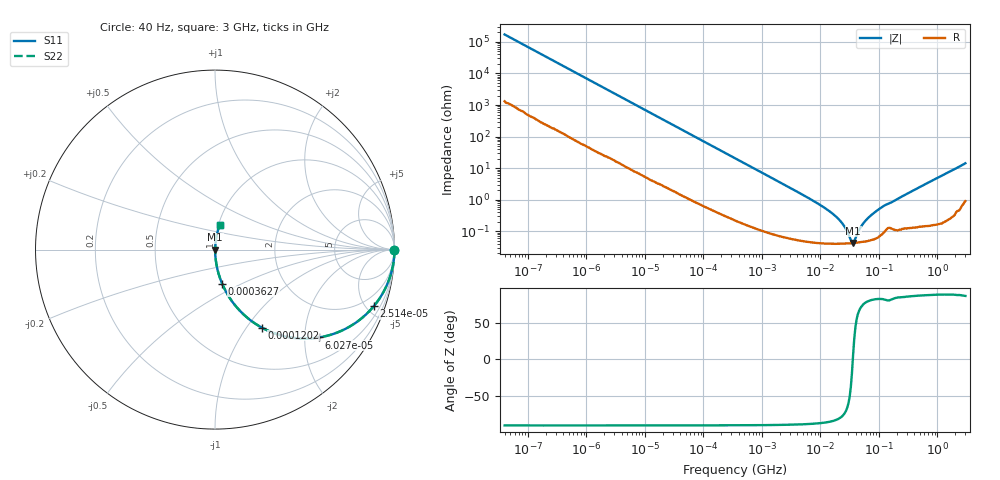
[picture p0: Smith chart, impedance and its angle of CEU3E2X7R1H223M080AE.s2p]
! S-parameter Generated by TDK Corporation
! Copyright(C) 2015 TDK Corporation.
! All Rights Reserved.
! TDK P/N: CEU3E2X7R1H223M080AE (Multilayer Ceramic Chip Capacitors)
! Property: C=22nF
! Size(LxWxT): 1.6x0.8x0.8mm, 0.063x0.031x0.031inches
! Model Type: s2p (Touchstone File Format Version 1.0)
! Frequency: DC=Yes Start=0.00004MHz Stop=3000MHz 396points Log-sweep
! Note: This model was converted from impedance.
! Model Generated on Jun. 23, 2015
! Hash(MD5):
! Port Assignments:
!  1 ---| |--- 2
! Applicable Conditions:
!  Temperature = 25 degC
!  DC Bias Voltage = 0 V
!  Small Signal Operation
! Terms and conditions regarding TDK Simulation Models
! (1)This simulation model is being provided solely for informational purposes. Please refer to the specifications of the products in terms of detailed characteristics of such products.
! (2)In no event shall TDK Corporation of any of its subsidiaries be liable for any loss or damage arising, directly or indirectly,
!  From any information contained in this simulation model, including, but not limited to loss or damages arising from any inaccuracies, omissions or errors in connection with such information.
! (3)Any and all copyrights on this simulation model are owned by TDK Corporation.
!  Duplication or redistribution of this simulation model without prior written permission from TDK Corporation is prohibited.
! (4)This simulation model is subject to any modification or change without any prior notice.
! (5)Neither TDK Corporation nor any of its subsidiaries shall make any warranty, express or implied,
!  Including but not limited to the correctness, implied warranties of merchantability and fitness for a particular purpose with respect to this simulation models.
! (6)The use of this simulation model shall be deemed to have consented to the terms and conditions hereof.
# MHz S MA R 50
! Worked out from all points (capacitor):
!   395 points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, 40 Hz to 3 GHz, reference 50 ohm
!   read as one part in series: C = 23.3 nF near 41.88 Hz
!   lowest |Z| = 43 mohm at 36.17 MHz (marker M1)
!   series resonance near 35.75 MHz, so ESL is about 850 pH
!   S11 on the Smith chart (normalised r, x): 40 Hz: open; 25.14 kHz: 1.05, -5.61; 60.27 kHz: 1.02, -2.35; 120.2 kHz: 1.01, -1.18; 362.7 kHz: 1.00, -0.39; 3 GHz: 1.02, +0.29
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4e-05  1 -0.0  0.0005836 89.5  0.0005836 89.5  1 -0.0
0.000834128  0.9998 -0.7  0.01202 88.9  0.01202 88.9  0.9998 -0.7
0.005256919  0.9966 -4.3  0.07484 85.3  0.07484 85.3  0.9966 -4.3
0.01739424  0.969 -13.9  0.2395 75.7  0.2395 75.7  0.969 -13.9
0.02513652  0.9395 -19.6  0.335 70.0  0.335 70.0  0.9395 -19.6
0.06026525  0.7585 -40.2  0.6453 49.3  0.6453 49.3  0.7585 -40.2
0.1201929  0.5071 -59.0  0.8573 30.5  0.8573 30.5  0.5071 -59.0
0.1994073  0.3358 -69.8  0.9387 19.6  0.9387 19.6  0.3358 -69.8
0.3464102  0.202 -77.7  0.9772 11.7  0.9772 11.7  0.202 -77.7
0.3627255  0.1933 -78.2  0.9791 11.1  0.9791 11.1  0.1933 -78.2
1.200196  0.05994 -85.7  0.9973 3.4  0.9973 3.4  0.05994 -85.7
7.22376  0.009705 -86.8  0.9995 0.6  0.9995 0.6  0.009705 -86.8
13.14015  0.004831 -84.9  0.9996 0.3  0.9996 0.3  0.004831 -84.9
20.81973  0.002351 -80.0  0.9996 0.1  0.9996 0.1  0.002351 -80.0
26.2067  0.001352 -72.3  0.9996 0.1  0.9996 0.1  0.001352 -72.3
34.54118  0.0004457 -18.5  0.9996 0.0  0.9996 0.0  0.0004457 -18.5
36.16801  0.00043 6.6  0.9996 -0.0  0.9996 -0.0  0.00043 6.6
45.52626  0.001092 65.8  0.9996 -0.1  0.9996 -0.1  0.001092 65.8
60.0049  0.002255 77.5  0.9995 -0.1  0.9995 -0.1  0.002255 77.5
95.07391  0.004714 82.1  0.9994 -0.3  0.9994 -0.3  0.004714 82.1
150.6385  0.007749 79.9  0.9987 -0.4  0.9987 -0.4  0.007749 79.9
3000  0.1404 78.3  0.9812 -8.1  0.9812 -8.1  0.1404 78.3
